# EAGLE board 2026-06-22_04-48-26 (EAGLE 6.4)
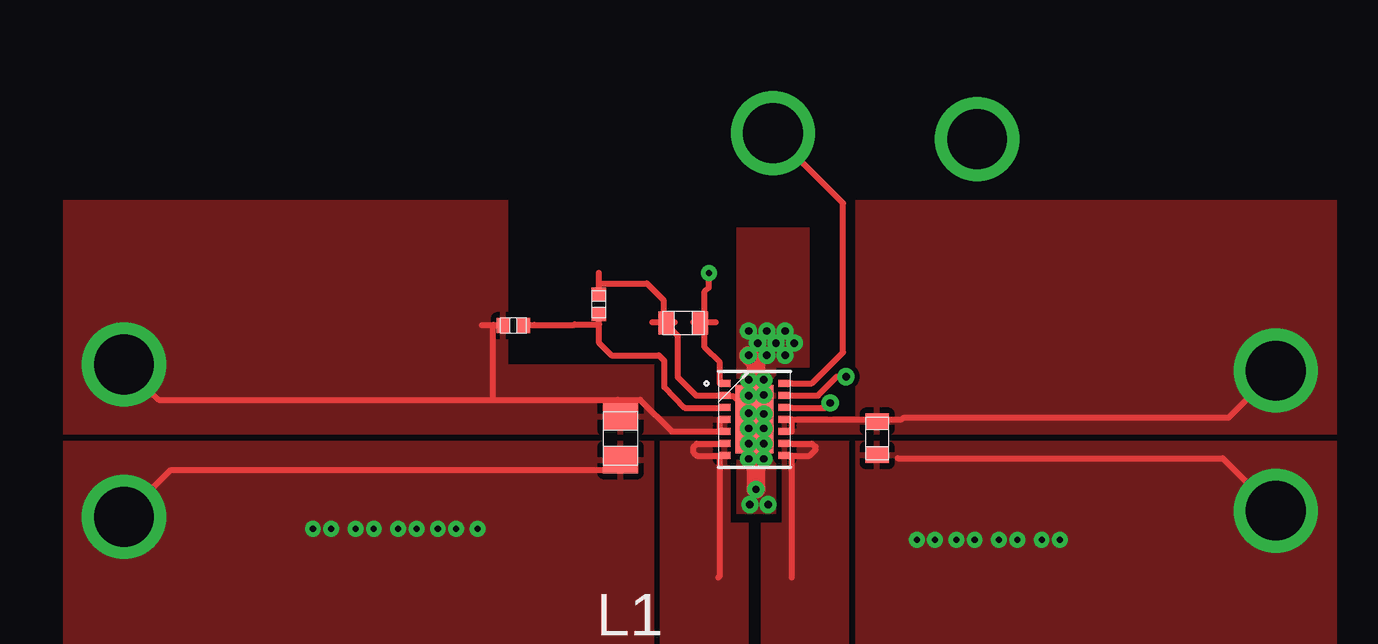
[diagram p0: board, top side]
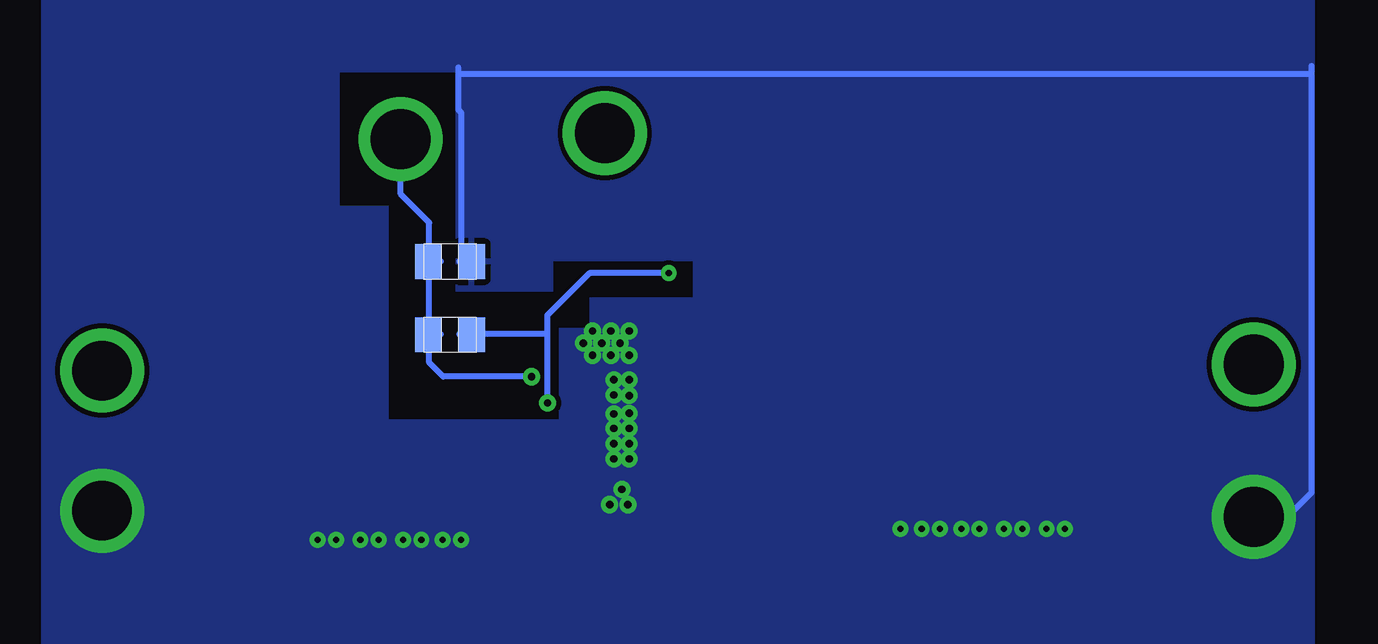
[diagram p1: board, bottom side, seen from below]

No outline drawn. Coordinates in mm, seen from the top.
Copper layers ((1*2)+(15*16)): TOP / INTERNAL1 / layer 15 / BOTTOM

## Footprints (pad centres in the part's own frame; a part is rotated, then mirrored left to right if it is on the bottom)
0603 = smd 0.66 x 0.965: 1 -0.699,0; 2 0.699,0
0805 = smd 1.118 x 1.448: 1 -0.902,0; 2 0.902,0
TP-1502 = drill 0.813 pad 1.651 round: 1 0,0
0402 = smd 0.559 x 0.61: 1 -0.419,0; 2 0.419,0
R-PVSON-N14 = smd 0.5 x 0.3: 1 -1.25,1.5; 2 -1.25,1; 3 -1.25,0.5; 4 -1.25,0; 5 -1.25,-0.5; 6 -1.25,-1; 7 -1.25,-1.5; 8 1.25,-1.5; 9 1.25,-1; 10 1.25,-0.5; 11 1.25,0; 12 1.25,0.5; 13 1.25,1; 14 1.25,1.5 | smd 1.58 x 2.85: 15 0,0

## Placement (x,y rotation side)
Cin  [0603]  60.1,51.03 270 top
Cout  [0805]  49.4,51.03 270 top
CvinA  [0603]  52.02,55.83 180 top
GND  [TP-1502]  76.68,47.98 0 top
GND1  [TP-1502]  28.68,47.73 0 top
Rfbb  [0402]  48.49,56.62 90 top
Rfbt  [0402]  44.93,55.73 0 top
RSync1  [0805]  62.2,58.39 0 bottom
RSync2  [0805]  62.2,55.35 180 bottom
TP_PG  [TP-1502]  55.73,63.73 0 top
TP_PS_SYNC  [TP-1502]  64.24,63.5 0 top
U1  [R-PVSON-N14]  54.99,51.82 0 top
Vin  [TP-1502]  76.68,53.85 0 top
Vout  [TP-1502]  28.68,54.08 0 top

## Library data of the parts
Cin = ultra-librarian; RefDes: Cin; Type: C1608X5R1A226M080AC
Cout = ultra-librarian; RefDes: Cout; Type: MSASJ21GBB5476MTNA01
CvinA = ultra-librarian; RefDes: CvinA; Type: EMK107B7104KA-T
GND = ultra-librarian; RefDes: GND; Type: TP-1502
GND1 = ultra-librarian; RefDes: GND1; Type: TP-1502
Rfbb = ultra-librarian; RefDes: Rfbb; Type: CRCW0402137KFKED
Rfbt = ultra-librarian; RefDes: Rfbt; Type: CRCW0402768KFKED
RSync1 = ultra-librarian; RefDes: RSync1; Type: ERJ-6ENF1373V
RSync2 = ultra-librarian; RefDes: RSync2; Type: ERJ-6ENF1373V
TP_PG = ultra-librarian; RefDes: TP_PG; Type: TP-1502
TP_PS_SYNC = ultra-librarian; RefDes: TP_PS_SYNC; Type: TP-1502
U1 = ultra-librarian; RefDes: U1; Type: TPS63020DSJR
Vin = ultra-librarian; RefDes: Vin; Type: TP-1502
Vout = ultra-librarian; RefDes: Vout; Type: TP-1502

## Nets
0: Cin.2 Cout.2 CvinA.2 GND1.1 GND.1 Rfbb.2 RSync1.1 RSync1.2 RSync2.2 TP_PS_SYNC.1 U1.2 U1.13 U1.15
1: Rfbb.1 Rfbt.2 U1.3
2: U1.8 U1.9
3: CvinA.1 RSync2.1 U1.1 U1.12
4: Cin.1 U1.10 U1.11 Vin.1
5: Cout.1 Rfbt.1 U1.4 U1.5 Vout.1
6: U1.6 U1.7
12: TP_PG.1 U1.14

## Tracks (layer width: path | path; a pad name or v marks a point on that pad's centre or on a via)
0  (via drill 0.25 pad 0.66, 0.3 pad 0.56, 2.49 pad 3.48)
  TOP 0.254: 48.51,57.48 50.49,57.48 51.21,56.77 51.21,55.88 51.79,55.3 51.79,53.57 52.55,52.81 53.54,52.81 53.57,52.78 54.1,52.78 55.04,51.84 55.04,51.82 | 56.54,52.81 57.63,52.81 58.42,53.59 v58.8,53.59 | v76.71,48.01 74.5,50.19 60.96,50.19 | v28.7,47.75 30.66,49.71 49.28,49.71 | 48.5,57 48.5,57.94 | 50.72,55.87 51.66,55.87
  TOP 0.762: 55.04,51.84 55.04,54.15 v54.74,54.48 | v55.04,48.9 55.04,51.82
  BOTTOM 0.254: 61.37,58.42 61.72,58.75 61.72,64.59 61.85,64.72 61.85,66.22 | v28.7,47.75 27.3,47.75 26.29,48.77 26.29,66.22 | 61.85,66.22 61.85,66.5 | 26.29,66.22 26.29,66.55 | v64.26,63.5 64.26,61.21 63.07,60.02 63.07,58.42 63.07,55.37 63.07,54.18 62.48,53.59 v58.8,53.59 | 26.29,66.22 61.85,66.22 | 62.59,55.36 63.52,55.36 | 62.59,58.41 63.52,58.41 | 60.88,58.41 61.82,58.41
  other vias: 36.58,47.24 38.35,47.24 40.89,47.24 40.13,47.24 42.55,47.24 54.79,48.26 54.74,50.8 54.74,50.16 54.74,52.81 55.12,54.99 56.64,54.99 56.26,54.48 62.51,46.79 65.18,46.79 66.95,46.79 54.74,53.47 54.74,52.07 54.74,51.44 54.74,55.5 56.26,55.5 37.34,47.24 39.12,47.24 41.78,47.24 43.43,47.24 55.55,48.26 55.37,50.8 55.37,50.16 55.37,52.83 55.88,54.99 55.5,54.48 64.16,46.79 63.4,46.79 67.72,46.79 65.94,46.79 61.75,46.79 55.37,53.47 55.37,52.04 55.37,51.44 55.5,55.5
  pour TOP (rank 6): 54.23,47.88 55.88,47.88 55.88,53.98 57.28,53.98 57.28,59.82 54.23,59.82
  pour TOP: 59.18,50.93 59.18,40.13 79.25,40.13 79.25,50.93
  pour TOP: 50.8,50.93 26.16,50.93 26.16,40.13 50.8,40.13
  pour BOTTOM (rank 5): 64.77,60.71 66.8,60.71 66.8,66.29 26.16,66.29 26.16,75.18 79.25,75.18 79.25,25.91 26.16,25.91 26.16,66.17 61.98,66.17 61.98,57.15 57.91,57.15 57.91,58.42 52.07,58.42 52.07,56.9 56.39,56.9 56.39,55.63 57.66,55.63 57.66,51.82 64.77,51.82
1
  TOP 0.254: 53.54,52.3 52.07,52.3 51.23,53.16 51.23,54.25 51,54.48 49.02,54.48 48.51,54.99 48.51,55.78 47.5,55.78 47.45,55.75 45.8,55.75 | 48.5,55.3 48.5,56.24 | 45.31,55.74 46.25,55.74
2
  TOP 0.254: 56.54,45.21 56.54,50.29 57.28,50.29 57.53,50.55 57.53,50.67 57.38,50.8 56.54,50.8 | 56.54,45.21
  pour TOP (rank 2): 56.13,50.93 58.93,50.93 58.93,40.13 55.24,40.13 55.24,47.5 56.13,47.5
3  (via drill 0.25 pad 0.56, 0.3 pad 0.56)
  TOP 0.254: v58.14,52.5 57.94,52.3 56.54,52.3 | 53.54,53.31 53.54,54.18 52.91,54.81 52.91,55.88 52.91,57.15 53.09,57.3 v53.09,57.91 | 52.43,55.87 53.37,55.87
  BOTTOM 0.254: v53.09,57.91 56.39,57.91 58.14,56.16 58.14,55.37 | 58.14,55.37 61.37,55.37 | v58.14,52.5 58.14,55.37 | 60.88,55.36 61.82,55.36
4  (via drill 2.49 pad 3.48)
  TOP 0.254: 63.5,51.89 | 63.5,51.89 61.21,51.89 61.11,51.82 56.54,51.82 56.54,51.31 | 63.5,51.89 74.75,51.89 v76.71,53.85
  pour TOP: 79.25,51.18 56.13,51.18 56.13,51.94 59.18,51.94 59.18,60.96 79.25,60.96
5  (via drill 2.49 pad 3.48)
  TOP 0.254: 53.54,51.82 53.54,51.31 51.54,51.31 50.22,52.63 49.28,52.63 44.12,52.63 | v28.7,54.1 30.15,52.63 44.12,52.63 | 44.12,52.63 44.09,52.63 44.09,55.75 | 43.61,55.74 44.55,55.74
  pour TOP (rank 4): 50.8,54.1 50.8,51.94 53.98,51.94 53.98,51.18 26.16,51.18 26.16,60.96 44.7,60.96 44.7,54.1
6
  TOP 0.254: 53.47,45.21 53.54,45.29 53.54,50.29 53.52,50.29 52.58,50.29 52.45,50.42 52.45,50.67 52.58,50.8 53.54,50.8
  pour TOP (rank 3): 53.98,50.93 51.05,50.93 51.05,40.13 54.74,40.13 54.74,47.5 53.98,47.5
12  (via drill 2.49 pad 3.48)
  TOP 0.254: v55.75,63.75 58.67,60.83 58.67,54.61 57.38,53.31 56.54,53.31

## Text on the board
ASSYNOTES: L1 | NOTE: | 1) Assemble only Rsync1 for Power save mode | option in Design and DNP Rsync2 | 2) Assemble only Rsync2 for FPWM mode | option in Design and DNP Rsync1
